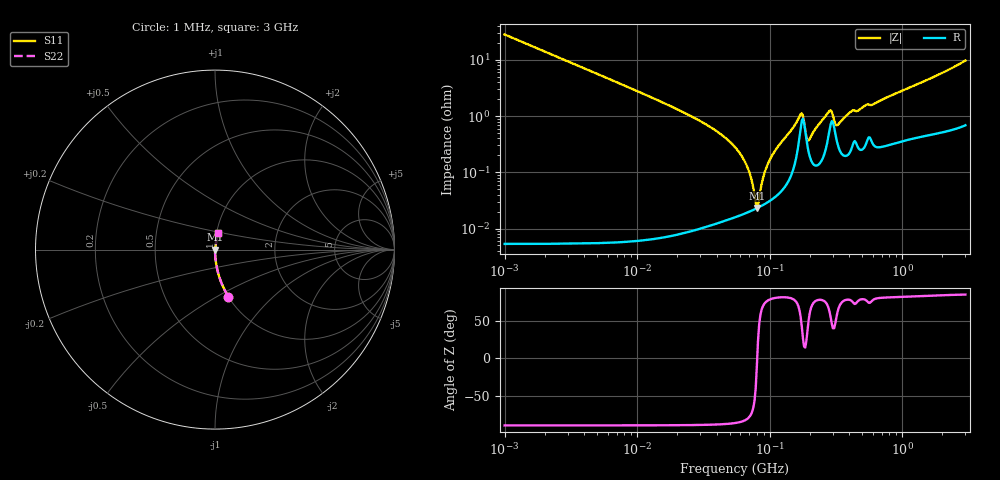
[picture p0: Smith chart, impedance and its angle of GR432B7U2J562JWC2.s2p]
!Murata Part Number: GR432B7U2J562JWC2
!These Parameters are Measured in Series Mode Connection
!Data Generated on Jun 10, 2025
!  o--ll--o
!Port1  Port2
!  o------o
!Operation Temp=25[degC], DC Bias Voltage=0[V]
!Freq. Start=1000[kHz] Stop=3[GHz] 401[Steps]
# Hz S RI R 50
!Freq.(Hz) S11(Real) S11(Imag) S21(Real) S21(Imag) S12(Real) S12(Imag) S22(Real) S22(Imag)
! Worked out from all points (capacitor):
!   401 points, 1 MHz to 3 GHz, reference 50 ohm
!   read as one part in series: C = 5.63 nF near 1.041 MHz
!   lowest |Z| = 23.3 mohm at 80.12 MHz (marker M1)
!   series resonance near 80.54 MHz, so ESL is about 690 pH
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1000000  0.074 -0.2617  0.926 0.2617  0.926 0.2617  0.074 -0.2617
3823119  0.00546 -0.0734  0.9945 0.0734  0.9945 0.0734  0.00546 -0.0734
1.461624e7  0.000417 -0.0187  0.9996 0.0187  0.9996 0.0187  0.000417 -0.0187
3.456417e7  0.000155 -0.00668  0.9998 0.00668  0.9998 0.00668  0.000155 -0.00668
5.477226e7  0.000166 -0.0028  0.9998 0.0028  0.9998 0.0028  0.000166 -0.0028
6.826239e7  0.000195 -0.00119  0.9998 0.00119  0.9998 0.00119  0.000195 -0.00119
7.248696e7  0.000206 -0.000757  0.9998 0.000757  0.9998 0.000757  0.000206 -0.000757
7.852918e7  0.000224 -0.000182  0.9998 0.000182  0.9998 0.000182  0.000224 -0.000182
8.011685e7  0.00023 -3.76e-05  0.9998 3.76e-05  0.9998 3.76e-05  0.00023 -3.76e-05
8.338914e7  0.000241 0.000253  0.9998 -0.000253  0.9998 -0.000253  0.000241 0.000253
9.216659e7  0.000275 0.000993  0.9997 -0.000993  0.9997 -0.000993  0.000275 0.000993
9.984923e7  0.00031 0.00161  0.9997 -0.00161  0.9997 -0.00161  0.00031 0.00161
1.680187e8  0.00431 0.00888  0.9957 -0.00888  0.9957 -0.00888  0.00431 0.00888
1.784169e8  0.00895 0.0045  0.991 -0.0045  0.991 -0.0045  0.00895 0.0045
1.93289e8  0.00285 0.0023  0.9972 -0.0023  0.9972 -0.0023  0.00285 0.0023
2.011837e8  0.00189 0.00351  0.9981 -0.00351  0.9981 -0.00351  0.00189 0.00351
2.094008e8  0.00151 0.00454  0.9985 -0.00454  0.9985 -0.00454  0.00151 0.00454
2.827291e8  0.00564 0.0109  0.9944 -0.0109  0.9944 -0.0109  0.00564 0.0109
3.252521e8  0.00324 0.00611  0.9968 -0.00611  0.9968 -0.00611  0.00324 0.00611
4.135554e8  0.00271 0.0118  0.9973 -0.0118  0.9973 -0.0118  0.00271 0.0118
8.005644e8  0.00355 0.0221  0.9965 -0.0221  0.9965 -0.0221  0.00355 0.0221
3e9  0.0159 0.0947  0.9841 -0.0947  0.9841 -0.0947  0.0159 0.0947
